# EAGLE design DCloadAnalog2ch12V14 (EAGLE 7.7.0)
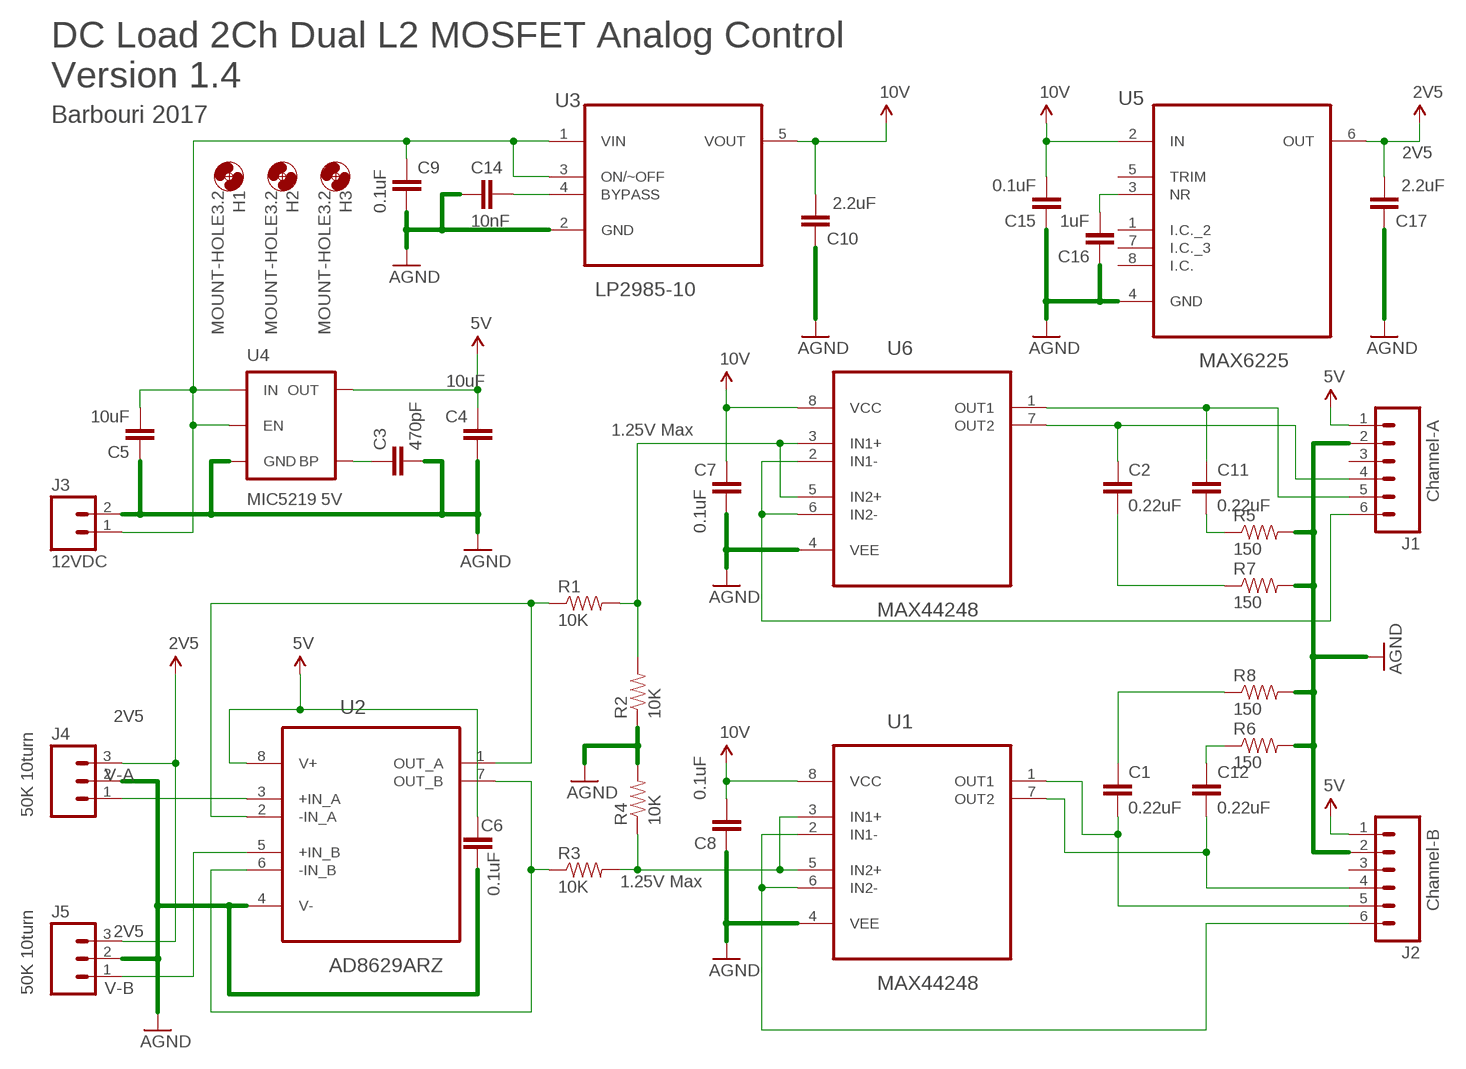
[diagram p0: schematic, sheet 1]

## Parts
C1  0.22uF  CAP0805  [0805]
C2  0.22uF  CAP0805  [0805]
C3  470pF  CAP0805  [0805]
C4  10uF  CAP0805  [0805]
C5  10uF  CAP0805  [0805]
C6  0.1uF  CAP0805  [0805]
C7  0.1uF  CAP0805  [0805]
C8  0.1uF  CAP0805  [0805]
C9  0.1uF  CAP0805  [0805]
C10  2.2uF  CAP0805  [0805]
C11  0.22uF  CAP0805  [0805]
C12  0.22uF  CAP0805  [0805]
C14  10nF  CAP0805  [0805]
C15  0.1uF  CAP0805  [0805]
C16  1uF  CAP0805  [0805]
C17  2.2uF  CAP0805  [0805]
H1  MOUNT-HOLE3.2  [3,2]
H2  MOUNT-HOLE3.2  [3,2]
H3  MOUNT-HOLE3.2  [3,2]
J1  Channel-A  M06LOCK  [1X06_LOCK]
J2  Channel-B  M06LOCK  [1X06_LOCK]
J3  12VDC  M023.5MM  [SCREWTERMINAL-3.5MM-2]
J4  M03LOCK  [1X03_LOCK]
J5  M03LOCK  [1X03_LOCK]
R1  10K  RESISTOR0805-RES  [0805]
R2  10K  RESISTOR0805-RES  [0805]
R3  10K  RESISTOR0805-RES  [0805]
R4  10K  RESISTOR0805-RES  [0805]
R5  150  RESISTOR0805-RES  [0805]
R6  150  RESISTOR0805-RES  [0805]
R7  150  RESISTOR0805-RES  [0805]
R8  150  RESISTOR0805-RES  [0805]
U1  MAX44248  MAX4126ESA+  [SOIC127P600X175-8N]
U2  AD8629ARZ  [SOIC127P600X175-8N]
U3  LP2985-10  LP2985-10DBVR  [SOT95P280X145-5N]
U4  MIC5219 5V  V_REG_MIC52195V  [SOT23-5]
U5  MAX6225  MAX6225ACSA+  [SOIC127P600X175-8N]
U6  MAX44248  MAX4126ESA+  [SOIC127P600X175-8N]

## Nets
2V5: C17.2 J4.3 J5.3 U5.6(OUT)
5V: C4.2 C6.2 J1.1 J2.1 U2.8(V+) U4.5(OUT)
10V: C7.2 C8.2 C10.2 C15.2 U1.8(VCC) U3.5(VOUT) U5.2(IN) U6.8(VCC)
AGND: C3.2 C4.1 C5.1 C6.1 C7.1 C8.1 C9.1 C10.1 C14.2 C15.1 C16.1 C17.1 J1.2 J2.2 J3.2 J4.2 J5.2 R2.1 R4.2 R5.2 R6.2 R7.2 R8.2 U1.4(VEE) U2.4(V-) U3.2(GND) U4.2(GND) U5.4(GND) U6.4(VEE)
N$1: R1.1 U2.1(OUT_A) U2.2(-IN_A)
N$2: R3.1 U2.6(-IN_B) U2.7(OUT_B)
N$5: C5.2 C9.2 J3.1 U3.1(VIN) U3.3(ON/~OFF) U4.1(IN) U4.3(EN)
N$6: R1.2 R2.2 U6.3(IN1+) U6.5(IN2+)
N$7: R3.2 R4.1 U1.3(IN1+) U1.5(IN2+)
N$8: C1.1 R8.1
N$9: J1.6 U6.2(IN1-) U6.6(IN2-)
N$10: J2.6 U1.2(IN1-) U1.6(IN2-)
N$11: C12.2 J2.4 U1.7(OUT2)
N$12: C11.1 J1.5 U6.1(OUT1)
N$13: C1.2 J2.5 U1.1(OUT1)
N$14: C11.2 R5.1
N$15: C12.1 R6.1
N$17: C3.1 U4.4(BP)
N$19: C14.1 U3.4(BYPASS)
N$20: C2.1 J1.4 U6.7(OUT2)
N$21: C2.2 R7.1
N$22: C16.2 U5.3(NR)
V-A: J4.1 U2.3(+IN_A)
V-B: J5.1 U2.5(+IN_B)
Unconnected: J1.3 J2.3 U5.1(I.C._2) U5.5(TRIM) U5.7(I.C._3) U5.8(I.C.)

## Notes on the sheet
- DC Load 2Ch Dual L2 MOSFET Analog Control
  Version 1.4
- Barbouri 2017
- 1.25V Max
- 50K 10turn
- 1.25V Max
- 50K 10turn

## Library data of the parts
C1-C12 C14-C17 = SparkFun-Capacitors:CAP: Capacitor
H1-H3 = holes:MOUNT-HOLE: MOUNTING HOLE with drill center marker
J1 J2 = SparkFun-Connectors:M06: Header 6 Standard 6-pin 0.1" header. Use with straight break away headers (SKU : PRT-00116), right angle break away headers (PRT-00553), swiss pins (PRT-00743), machine pins (PRT-00117), and female headers (PRT-00115). Molex polarized connector foot print use with SKU : PRT-08094 with associated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
J3 = SparkFun-Connectors:M02: Standard 2-pin 0.1" header. Use with; PROD_ID: CONN-08399
J4 J5 = SparkFun-Connectors:M03: Header 3 Standard 3-pin 0.1" header. Use with straight break away headers (SKU : PRT-00116), right angle break away headers (PRT-00553), swiss pins (PRT-00743), machine pins (PRT-00117), and female headers (PRT-00115). Molex polarized connector foot print use with SKU : PRT-08232 with associated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
R1-R8 = SparkFun-Resistors:RESISTOR: Resistor
U1 U6 = Maxim_By_element14_Batch_1:MAX4126ESA+: Single/Dual/Quad, Wide-Bandwidth, Low-Power, Single-Supply Rail-to-Rail I/O Op Amps; MPN: MAX4126ESA+; OC_FARNELL: 1422317; OC_NEWARK: 23K5945; PACKAGE: SOIC-8; SUPPLIER: Maxim
U2 = Analog Devices_By_element14_Batch_1:AD8629ARZ: Zero-Drift, Single-Supply, Rail-to-Rail Input/Output Operational Amplifier; MPN: AD8629ARZ; OC_FARNELL: 9994300; OC_NEWARK: 19M0981; PACKAGE: SOIC-8; SUPPLIER: Analog Devices
U3 = Texas Instruments_By_element14_Batch_1:LP2985-10DBVR: LOW-DROPOUT REGULATOR WITH SHUTDOWN; MPN: LP2985-10DBVR; OC_FARNELL: -; OC_NEWARK: 24R9588; PACKAGE: SOT-23-5; SUPPLIER: Texas Instruments
U4 = SparkFun-PowerIC:V_REG_MIC5219: V_REG MIC5219 Standard 3.3V and 5V 500mA LDO voltage regulator in SOT-23 layout. Micrel part MIC5219. BP (by-pass) pin is used to lower output noise with 470pF cap, may be left open.; PROD_ID: VREG-10107
U5 = Maxim_By_element14_Batch_1:MAX6225ACSA+: Low-Noise, Precision, +2.5V/+4.096V/+5V Voltage References; MPN: MAX6225ACSA+; OC_FARNELL: -; OC_NEWARK: 59J3522; PACKAGE: SOIC-8; SUPPLIER: Maxim

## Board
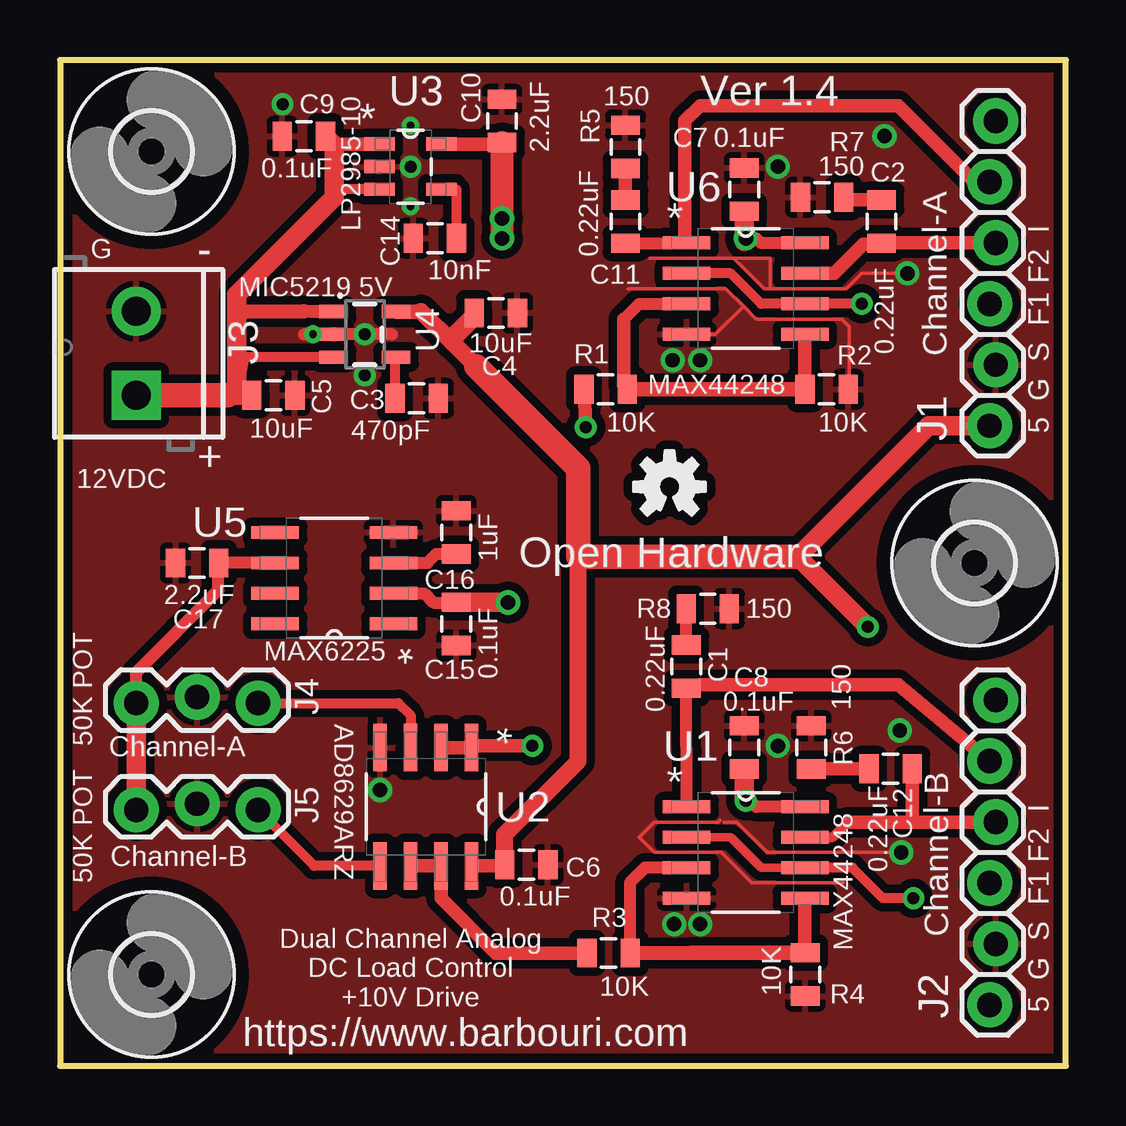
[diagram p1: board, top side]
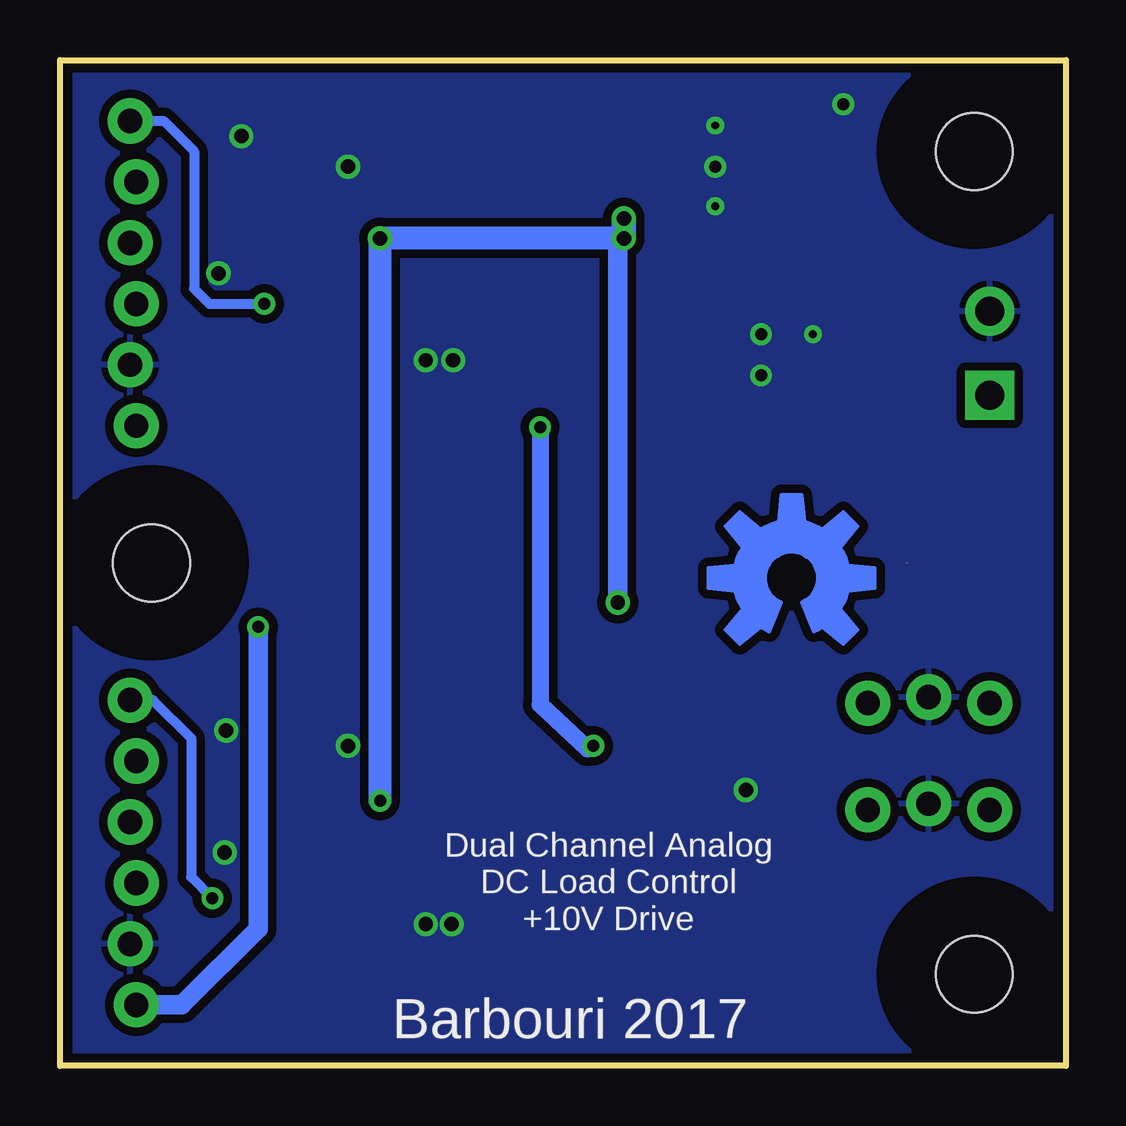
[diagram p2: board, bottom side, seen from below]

Size 41.91 x 41.91 mm. Coordinates in mm from the lower left corner, seen from the top.
Outline: 0,0 41.91,0 41.91,41.91 0,41.91 0,0
Copper layers (1*16): Top 0.035mm / dielectric 1.5mm / Bottom 0.035mm
Design rules "default *": minimum track width 6mil, minimum drill 10mil, track to track 14mil, track to pad 14mil, pad to pad 14mil, via to via 14mil, smd to smd 8mil, copper to edge 15mil, drill to drill 8mil, minimum pad ring 10mil, minimum via ring 8mil, stop-mask expansion 4mil, vias tented up to drill 0mil, thermal gap 10mil

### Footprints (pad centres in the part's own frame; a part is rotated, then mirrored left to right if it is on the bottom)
0805 = smd 0.8 x 1.2: 1 -0.9,0; 2 0.9,0
3,2 = hole 3.2: 0,0
1X06_LOCK = drill 1.016 pad 1.88: 1 0,0; 2 2.54,-0.254; 3 5.08,0; 4 7.62,-0.254; 5 10.16,0; 6 12.7,-0.254
SCREWTERMINAL-3.5MM-2 = drill 1.2 pad 2.032 square: 1 0,0 | drill 1.2 pad 2.032: 2 3.5,0
1X03_LOCK = drill 1.016 pad 1.88: 1 0,0.127; 2 2.54,-0.127; 3 5.08,0.127
SOIC127P600X175-8N = smd 1.981 x 0.533: 1 -2.464,1.905; 2 -2.464,0.635; 3 -2.464,-0.635; 4 -2.464,-1.905; 5 2.464,-1.905; 6 2.464,-0.635; 7 2.464,0.635; 8 2.464,1.905
SOIC127P600X175-8N' = smd 1.981 x 0.559: 1 -2.464,1.905; 2 -2.464,0.635; 3 -2.464,-0.635; 4 -2.464,-1.905; 5 2.464,-1.905; 6 2.464,-0.635; 7 2.464,0.635; 8 2.464,1.905
SOT95P280X145-5N = smd 1.27 x 0.559: 1 -1.295,0.94; 2 -1.295,0; 3 -1.295,-0.94; 4 1.295,-0.94; 5 1.295,0.94
SOT23-5 = smd 0.55 x 1.2: 1 -0.95,-1.3; 2 0,-1.3; 3 0.95,-1.3; 4 0.95,1.3; 5 -0.95,1.3

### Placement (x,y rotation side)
C1  26.1,16.64 270 top
C2  34.23,35.18 90 top
C3  14.86,27.81 0 top
C4  18.16,31.37 180 top
C5  8.89,27.94 180 top
C6  19.43,8.38 180 top
C7  28.51,36.51 270 top
C8  28.51,13.27 270 top
C9  10.16,38.73 0 top
C10  18.41,39.37 270 top
C11  23.56,35.18 90 top
C12  34.61,12.38 0 top
C14  15.62,34.48 180 top
C15  16.51,18.41 90 top
C16  16.51,22.23 270 top
C17  5.71,20.95 0 top
H1  3.81,3.81 0 top
H2  3.81,38.1 0 top
H3  38.1,20.95 0 top
J1  38.73,26.67 90 top
J2  38.73,2.54 90 top
J3  3.17,27.94 90 top
J4  8.26,15.24 180 top
J5  8.26,10.79 180 top
R1  22.73,28.19 0 top
R2  31.94,28.19 180 top
R3  22.86,4.7 0 top
R4  31.05,3.81 270 top
R5  23.56,38.29 90 top
R6  31.31,13.27 90 top
R7  31.75,36.2 180 top
R8  26.99,19.05 0 top
U1  28.57,8.89 0 top
U2  AD8629ARZ  [SOIC127P600X175-8N']  15.24,10.79 270 top
U3  14.61,37.47 0 top
U4  12.7,30.48 270 top
U5  11.43,20.32 180 top
U6  28.57,32.38 0 top
U$10  [OSHW-LOGO-L_COPPER]  11.43,20.32 0 bottom
U$11  [OSHW-LOGO-S_COPPER]  25.4,24.13 0 top
U$12  [OSHW-LOGO-S]  25.4,24.13 0 top

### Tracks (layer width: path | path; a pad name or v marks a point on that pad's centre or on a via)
2V5  (1 unrouted)
  Top 0.508: J4.3 3.17,16.38 6.6,19.81 6.6,20.94 | U5.6 C17.2
  Top 0.813: J5.3 J4.3
5V  (via drill 0.5)
  Top 0.559: U2.8 18.48,8.33
  Top 0.61: U4.5 15.05,31.43 | 16.51,30.48 16.32,30.16 | 18.48,8.33 C6.2
  Top 0.711: 15.05,31.43 16.32,30.16 17.34,29.15 17.78,28.7 | C6.2 18.53,9.64 21.59,12.7 21.59,21.21
  Top 0.813: J1.1 36.2,26.67 30.73,21.21 v33.66,18.29 | C4.2 17.26,31.23 16.51,30.48
  Top 1.016: 17.34,29.15 21.59,24.89 21.59,21.21 30.73,21.21
  Bottom 0.813: v33.66,18.29 33.66,5.71 36.83,2.54 J2.1
10V  (via drill 0.5, 0.6)
  Top 0.406: 16.5,19.3 C15.2
  Top 0.508: U1.8 29.02,10.79 28.77,11.05 v28.57,11.05 | v28.57,34.48 29.02,34.48 29.21,34.29 U6.8 | 18.35,38.41 C10.2 | U5.2 15.18,19.68 15.56,19.3 16.5,19.3 | 18.66,19.32 v18.67,19.3
  Top 0.559: U3.5 18.35,38.41
  Top 0.813: C8.2 28.51,11.05 v28.57,11.05 | C7.2 28.51,34.35 v28.57,34.48 | C15.2 18.66,19.32
  Top 0.965: C10.2 v18.41,34.48
  Bottom 0.508: 18.67,34.23 v18.41,34.48
  Bottom 0.813: v18.67,19.3 18.67,34.23
  Bottom 0.965: v28.57,11.05 v28.57,34.48 v18.41,34.48
  Bottom 1.016: v18.41,35.31 v18.41,34.48
AGND  (via drill 0.33, 0.5, 0.6)
  Top 0.152: v35.05,8.89 29.46,8.89 28.19,10.16 27.69,10.16 | 32.64,7.62 28.83,7.62 27.56,8.89 24.77,8.89 24.13,9.53 24.77,10.16 27.43,10.16 27.5,10.22 | 29.59,32.38 32.77,32.38 33.4,33.02 v35.31,33.02 | 29.59,32.38 29.34,32.38 28.07,33.66 | 28.07,33.66 24.57,33.66 | 28.48,31.66 29.02,31.11 32.58,31.11 32.89,30.8 32.89,28.26 | 28.48,31.66 27.75,32.38 23.69,32.38 | U6.4 27.3,30.48 28.48,31.66 | 29.59,32.38 29.59,33.66 28.07,33.66
  Top 0.508: 13.84,30.48 10.16,30.48
  other vias: 10.54,30.48 12.7,30.48 12.7,28.77 9.27,40.07 34.99,13.97 29.91,13.34 26.67,29.4 34.35,38.73 29.91,37.47 26.67,5.91 14.61,37.47 14.61,35.81 14.61,39.18 25.53,29.4 25.59,5.91 13.34,11.49
  pour Top: 0,0 41.91,0 41.91,41.91 0,41.91
  pour Bottom: 0,0 41.91,0 41.91,41.91 0,41.91
N$1  (via drill 0.5)
  Top 0.508: R1.1 21.84,28.19 | 17.22,13.34 U2.1
  Top 0.559: 21.84,28.19 v21.91,26.61 | v19.68,13.34 17.22,13.34 | U2.2 U2.1
  Bottom 0.508: 19.94,13.21 19.81,13.21 v19.68,13.34
  Bottom 0.711: v21.91,26.61 21.91,15.05 19.94,13.21
N$2
  Top 0.559: R3.1 18.16,4.7 15.88,6.99 U2.7 U2.6
N$5
  Top 0.406: U4.3 7.67,29.53 7.36,27.94 | U3.3 11.73,36.52 11.43,36.83
  Top 0.508: 11.73,38.41 11.43,38.1
  Top 0.533: U4.1 10.48,31.43 10.16,31.43
  Top 0.559: U3.1 11.73,38.41
  Top 0.61: 10.16,31.43 7.67,31.43 7.36,31.11
  Top 0.813: 6.99,27.94 7.36,27.94 | C5.2 7.36,27.94 | 7.36,27.94 7.36,31.11 7.36,32.12 11.43,36.2 11.43,36.83 11.43,38.1 11.43,38.37 C9.2
  Top 1.016: J3.1 6.99,27.94
N$6
  Top 0.406: 23.5,28.33 R1.2 | R2.2
  Top 0.508: 23.5,31.11 24.13,31.75 U6.3
  Top 0.559: 23.5,31.11 23.5,28.33 | U6.5 R2.2
  Top 0.61: R1.2 R2.2
N$7
  Top 0.508: 31.04,4.72 R4.1 | U1.3 24.38,8.26 23.75,7.62 23.75,4.71 R3.2
  Top 0.559: U1.5 31.04,4.72
  Top 0.61: R4.1 26.31,4.71 R3.2
N$8
  Top 0.508: C1.1 R8.1
N$9  (via drill 0.5)
  Top 0.406: U6.2 27.94,33.02 29.21,31.75 U6.6 v33.4,31.75
  Bottom 0.406: J1.6 37.59,39.37 36.32,38.1 36.32,32.38 35.69,31.75 v33.4,31.75
N$10  (via drill 0.5)
  Top 0.356: U1.2 27.94,9.53 29.21,8.26 U1.6
  Top 0.406: v35.56,6.99 34.29,6.99 33.02,8.26 U1.6
  Bottom 0.406: J2.6 38.04,15.24 36.45,13.65 36.45,7.87 v35.56,6.99
N$11
  Top 0.406: U1.7 32.19,9.53 32.83,10.16
  Top 0.508: 35.51,10.21 35.62,10.16
  Top 0.559: 32.83,10.16 35.62,10.16 J2.4 | C12.2 35.51,10.21
N$12
  Top 0.406: U6.1 26.04,34.37 | J1.5 38.1,36.83
  Top 0.508: C11.1 U6.1
  Top 0.559: 38.1,36.83 34.92,40.01 26.67,40.01 26.04,39.37 26.04,34.37
N$13
  Top 0.508: 26.67,15.88 C1.2 U1.1
  Top 0.559: J2.5 34.92,15.88 26.67,15.88
N$14
  Top 0.559: C11.2 R5.1
N$15
  Top 0.559: C12.1 31.81,12.38 31.8,12.37 R6.1
N$17
  Top 0.406: C3.1 13.96,29.49 U4.4
N$19
  Top 0.406: C14.1 16.52,36.51 U3.4
N$20
  Top 0.406: C2.1 34.17,34.23
  Top 0.559: J1.4 C2.1 | U6.7 32.26,33.02 33.47,34.23 34.17,34.23
N$21
  Top 0.406: 32.77,36.08 R7.1
  Top 0.559: C2.2 32.77,36.08
N$22
  Top 0.406: 16.5,21.34 C16.2
  Top 0.508: U5.3 15.3,20.95 15.68,21.34 16.5,21.34
V-A
  Top 0.406: J4.1 14.1,15.11 14.61,14.61 U2.3
V-B
  Top 0.406: U2.5 10.59,8.33 J5.1

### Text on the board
tNames: Ver 1.4 | G | - | 5 G S F1 F2 I | + | Open Hardware | 50K POT | Channel-A | 50K POT | Channel-B | Dual Channel Analog / DC Load Control / +10V Drive | 5 G S F1 F2 I | https://www.barbouri.com
bNames: Dual Channel Analog / DC Load Control / +10V Drive | Barbouri 2017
